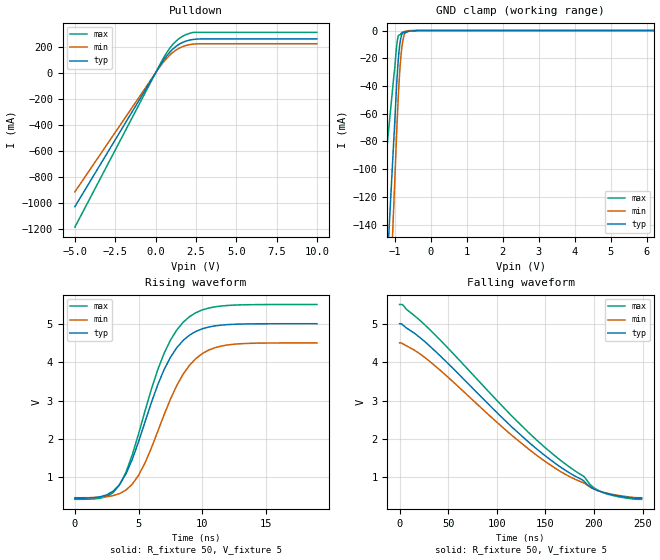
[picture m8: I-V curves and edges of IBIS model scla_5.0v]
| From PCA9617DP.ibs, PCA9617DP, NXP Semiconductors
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[Model]   scla_5.0v
Model_type Open_drain
Vref=5.000E+00
Rref=1.350E+03
Cref=5.000E-11
Vmeas=2.500E+00
C_comp   9.000E-13   8.790E-13   9.210E-13
[Voltage Range]   5.000E+00   4.500E+00   5.500E+00
[POWER Clamp Reference]   5.000E+00   4.500E+00   5.500E+00
[GND Clamp Reference]   0.000E+00   0.000E+00   0.000E+00
[Pullup Reference]   5.000E+00   4.500E+00   5.500E+00
[Pulldown Reference]   0.000E+00   0.000E+00   0.000E+00
[Temperature Range]   25   85   -40
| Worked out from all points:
|   slope of the pulldown table from 0 to 0.75 V, typ, clamps not added: 5.35 ohm
|   GND clamp passes 1 mA (typ) near -0.65 V on its own axis
|   rising waveform, R_fixture 50, V_fixture 5: 20-80 % time 3.08ns typ, 3.17ns min, 3.03ns max; typ from 0.456 V to 5 V
|   falling waveform, R_fixture 50, V_fixture 5: 20-80 % time 115ns typ, 112ns min, 120ns max; typ from 5 V to 0.456 V
[GND Clamp]
-5V       -2.033A    -2.678A    -1.095A
-1.02V    -76.43mA   -122.4mA   -32.01mA
-940mV    -36.59mA   -70.69mA   -10.08mA
-900mV    -20.96mA   -47.85mA   -3.695mA
-860mV    -10.45mA   -29.66mA   -3.084mA
-840mV    -6.955mA   -22.48mA   -2.944mA
-820mV    -4.424mA   -16.57mA   -1.945mA
-780mV    -1.587mA   -8.169mA   -1.012mA
-740mV    -1.516mA   -3.381mA   -868.1uA
-700mV    -1.48mA    -1.012mA   -530.8uA
-600mV    -460.9uA   -137.9uA   -125uA
10V       0A         0A         0A
[Pulldown]
-5V       -1.026A    -912mA     -1.183A
360mV     72.79mA    62.73mA    85.83mA
600mV     116.6mA    100.3mA    138.1mA
900mV     161.9mA    139.4mA    192.8mA
1.42V     217mA      187.1mA    260.2mA
1.9V      245mA      211.3mA    295.3mA
2.36V     257.4mA    221.8mA    311.4mA
10V       261.2mA    224.5mA    311.9mA
[Rising Waveform]
R_fixture = 50
V_fixture = 5
V_fixture_min = 4.5
V_fixture_max = 5.5
0s        455.9mV    470.6mV    428.7mV
2.5ns     544.5mV    497.7mV    502.6mV
3.5ns     811mV      576.3mV    800.4mV
4ns       1.084V     667.7mV    1.126V
5ns       1.929V     1.055V     2.133V
7ns       3.802V     2.628V     4.226V
8ns       4.376V     3.393V     4.838V
9ns       4.703V     3.919V     5.184V
11.5ns    4.964V     4.419V     5.461V
19ns      5V         4.5V       5.5V
[Falling Waveform]
R_fixture = 50
V_fixture = 5
V_fixture_min = 4.5
V_fixture_max = 5.5
0s        5V         4.5V       5.5V
3.5ns     4.965V     4.475V     5.486V
30.5ns    4.43V      4.029V     4.86V
115.5ns   2.311V     2.094V     2.596V
160ns     1.367V     1.24V      1.557V
190ns     893.8mV    850.5mV    1.016V
197ns     740.8mV    732.1mV    790.1mV
205ns     644.8mV    648.4mV    653.6mV
223.5ns   524.3mV    536.9mV    504.4mV
249ns     455.9mV    470.6mV    428.7mV
[Ramp]
dV/dt_r   2.7265E+00/3.0610E-09   2.4176E+00/3.1520E-09   3.0428E+00/3.0050E-09
dV/dt_f   2.7265E+00/1.1544E-07   2.4176E+00/1.1179E-07   3.0428E+00/1.2044E-07
R_load = 50
